PROGRAM Tc3_DALI_Test
VAR
	nStep						:	INT;
	fbTon						:	TON;
	fbOff						:	FB_DALI102Off(Communication.fbKL6821CommunicationTc3);
	fbGetInputNotification		:	FB_DALIGetInputNotification(Communication.fbKL6821CommunicationTc3);
	nRisingEdge					:	INT;
	nFallingEdge				:	INT;	
END_VAR

CASE nStep OF
0:
	fbTon(IN := TRUE, PT := T#500MS);		
	IF (fbTon.Q) THEN
		fbTon(IN := FALSE);
		fbOff(bStart := FALSE);
		nStep := 10;
	END_IF

10:
	fbOff(	bStart := TRUE,
			nAddress := 0,
			eCommandPriority := E_DALICommandPriority.MiddleLow);
	IF (NOT fbOff.bBusy) THEN
		fbOff(bStart := FALSE);
		nStep := 0;
	END_IF
ELSE
	fbOff(bStart := FALSE);
	fbTon(IN := FALSE);
	nStep := 0;
END_CASE

fbGetInputNotification(	bEnable := TRUE,
						eEventScheme := E_DALIEventScheme.DeviceInstance,
						nAddressInfo1 := 3,
						nAddressInfo2 := 0);
IF (NOT fbGetInputNotification.bError) THEN
	IF (fbGetInputNotification.bNewData) THEN
		IF (fbGetInputNotification.nEventInfo = 16#0001) THEN // Button pushed		
			nRisingEdge := nRisingEdge + 1;
		END_IF
		IF (fbGetInputNotification.nEventInfo = 16#0000) THEN // Button released
			nFallingEdge := nFallingEdge + 1;
		END_IF
	END_IF
END_IF

END_PROGRAM
